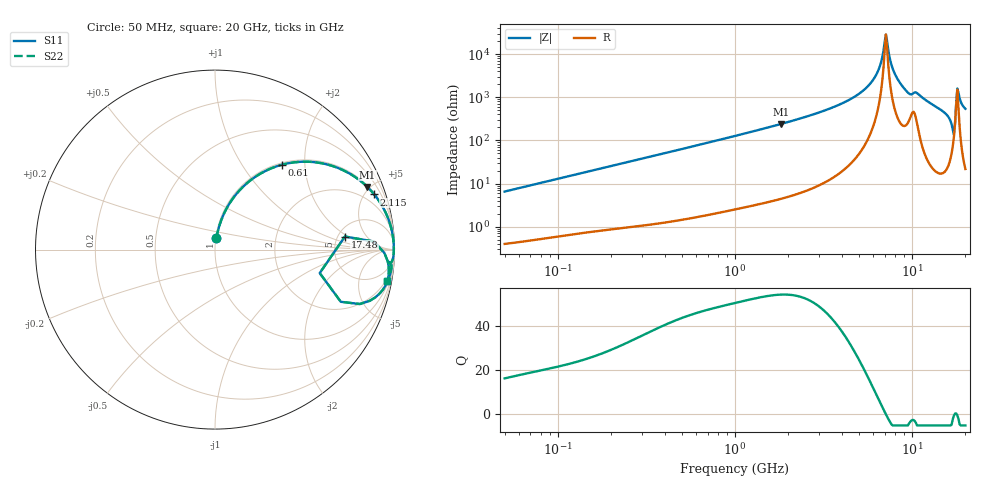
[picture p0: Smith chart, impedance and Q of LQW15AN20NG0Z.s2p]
!Murata Part Number: LQW15AN20NG0Z
!These Parameters are Measured in Series Mode Connection
!  o--[Z]--o
!Port1  Port2
!  o-------o
!Freq. Start=50[MHz] Stop=20[GHz], 401[Steps]
# Hz S RI R 50
!Freq.(Hz) S11(Real) S11(Imag) S21(Real) S21(Imag) S12(Real) S12(Imag) S22(Real) S22(Imag)
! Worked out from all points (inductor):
!   401 points, 50 MHz to 20 GHz, reference 50 ohm
!   read as one part in series: L = 20.7 nH near 51.52 MHz
!   highest Q = 54.3 at 1.821 GHz (marker M1), where L = 21.1 nH
!   self-resonance near 7.115 GHz
!   S11 on the Smith chart (normalised r, x): 50 MHz: 1.01, +0.13; 610 MHz: 1.03, +1.54; 2.115 GHz: 1.11, +5.73; 17.48 GHz: 5.78, +1.79; 20 GHz: 1, -11
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5e7  0.00819 0.0646  0.9918 -0.0646  0.9918 -0.0646  0.00819 0.0646
1.364002e8  0.0361 0.1671  0.9639 -0.1671  0.9639 -0.1671  0.0361 0.1671
3.721004e8  0.1871 0.3775  0.8129 -0.3775  0.8129 -0.3775  0.1871 0.3775
6.100003e8  0.375 0.4734  0.625 -0.4734  0.625 -0.4734  0.375 0.4734
1e9  0.6157 0.4766  0.3843 -0.4766  0.3843 -0.4766  0.6157 0.4766
1.820564e9  0.8487 0.3492  0.1513 -0.3492  0.1513 -0.3492  0.8487 0.3492
2.114743e9  0.8871 0.3074  0.1129 -0.3074  0.1129 -0.3074  0.8871 0.3074
2.728004e9  0.9354 0.2362  0.0646 -0.2362  0.0646 -0.2362  0.9354 0.2362
5.194772e9  0.9913 0.0734  0.00874 -0.0734  0.00874 -0.0734  0.9913 0.0734
6.311513e9  0.9959 0.0282  0.00407 -0.0282  0.00407 -0.0282  0.9959 0.0282
6.601595e9  0.9964 0.0177  0.00364 -0.0177  0.00364 -0.0177  0.9964 0.0177
7.009217e9  0.9965 0.0037  0.00345 -0.0037  0.00345 -0.0037  0.9965 0.0037
7.222371e9  0.9965 -0.0034  0.00355 0.0034  0.00355 0.0034  0.9965 -0.0034
7.442007e9  0.9962 -0.0106  0.00378 0.0106  0.00378 0.0106  0.9962 -0.0106
8.141811e9  0.9944 -0.0328  0.00557 0.0328  0.00557 0.0328  0.9944 -0.0328
9.457416e9  0.9797 -0.0732  0.0203 0.0732  0.0203 0.0732  0.9797 -0.0732
1.066139e10  0.9786 -0.0754  0.0214 0.0754  0.0214 0.0754  0.9786 -0.0754
1.504638e10  0.9479 -0.2038  0.0521 0.2038  0.0521 0.2038  0.9479 -0.2038
1.670968e10  0.8066 -0.3032  0.1934 0.3032  0.1934 0.3032  0.8066 -0.3032
1.747767e10  0.724 0.0728  0.276 -0.0728  0.276 -0.0728  0.724 0.0728
1.828096e10  0.9625 -0.0653  0.0375 0.0653  0.0375 0.0653  0.9625 -0.0653
2e10  0.9605 -0.1757  0.0395 0.1757  0.0395 0.1757  0.9605 -0.1757
